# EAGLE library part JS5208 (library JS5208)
E-SWITCH - JS5208 - SWITCH, NAVIGATION, 5 POSITION, 20mA, SMD Source: Datasheet
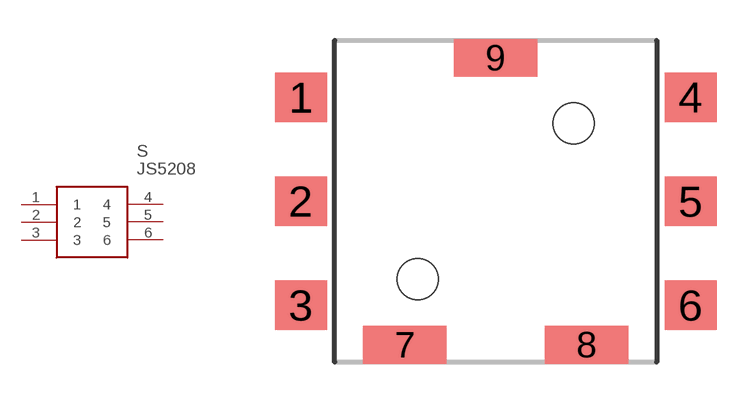
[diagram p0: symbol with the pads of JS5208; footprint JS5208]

Designator prefix S

## JS5208 (Description: E-SWITCH - JS5208 - SWITCH, NAVIGATION, 5 POSITION, 20mA, SMD; Height: mm; Manufacturer_Name: E-Switch; Manufacturer_Part_Number: JS5208; Mouser_Part_Number: 612-JS5208; Mouser_Price-Stock: https://www.mouser.com/Search/Refine.aspx?Keyword=612-JS5208)  [JS5208]
1  1
2  2
3  3
4  4
5  5
6  6

## Footprint JS5208 (pad centres in mm)
JS5208
smd 2 x 1.9: 1 -7.5,4; 2 -7.5,0; 3 -7.5,-4; 4 7.5,4; 5 7.5,0; 6 7.5,-4
smd 3.2 x 1.45: 7 -3.5,-5.525; 8 3.5,-5.525; 9 0,5.525
hole 1.6 at 3,3
hole 1.6 at -3,-3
